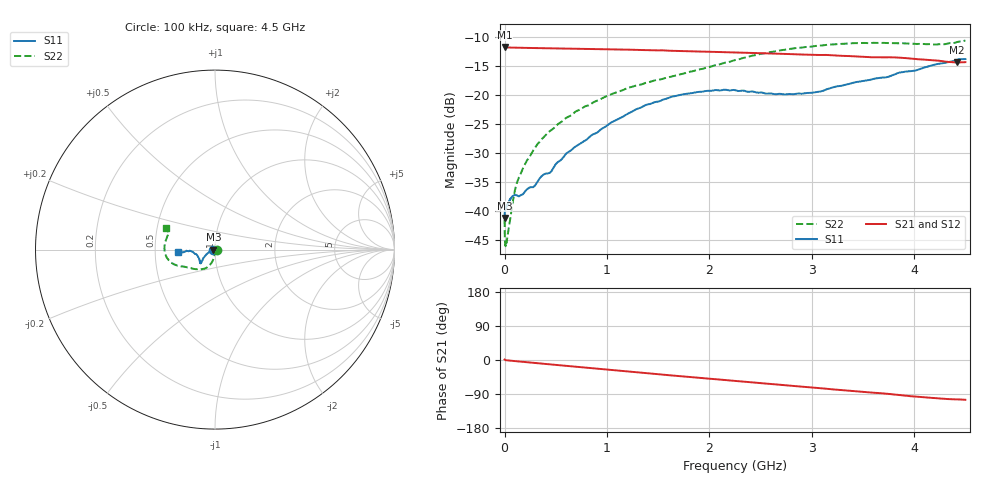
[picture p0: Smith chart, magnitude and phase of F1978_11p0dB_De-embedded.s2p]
! Integrated Device Technology
! Corporate Headquarters
! 6024 Silver Creek Valley Road
! San Jose, CA 95138  USA
! Phone:  1-408-284-8200
! Toll Free:  1-800-223-1366
! Webpage:  http://www.idt.com/
! Timing and RF Division
! 515 Groton Road, Suite 102
! Westford, MA 01886-6024
! Device:  F1978
! Description: 6-bit, 75 ohm, 0.5 dB Digital Step Attenuator
! Frequency:  5.0 MHz -  3.00 GHz
! Package:  4x4 mm QFN Plastic Package: 20 pin
! Ports:  2 RF, 11 DC
!  Pin  1  = D5 (16 dB)
!  Pin  2  = RF1  =  Port 1
!  Pin  3  = Serial Data In (DATA)
!  Pin  4  = Serial Clock (CLK)
!  Pin  5  = Serial Latch Enable (LE)
!  Pin  6  = VDD
!  Pin  7  = NC
!  Pin  8  = NC
!  Pin  9  = NC
!  Pin 10  = GND
!  Pin 11  = GND
!  Pin 12  = NC
!  Pin 13  = VMODE
!  Pin 14  = RF2  =  Port 2
!  Pin 15  = D4 (8 dB)
!  Pin 16  = D3 (4 dB)
!  Pin 17  = D2 (2 dB)
!  Pin 18  = NC
!  Pin 19  = D1 (1 dB)
!  Pin 20  = D0 (0.5 dB)
! State:  22
! Atten State:  11.0 dB
! Voltage:  +3.30 Volts
! Current:  0.592 mA
! Data:  The device was measured on a F1975 evaluation board which has
!  individual transmission lines to the RF pins.  Data was collected
!  using a calibrated network analyzer.  The evaluation board was
!  de-embedded using Automatic Fixture Removal (AFR).
!  The reference plane is the edge of the package pin.
! Misc:
!  Action Tracker AT0416
! Date Measured:  2018-02-08
! Date:  2018-03-26  MJV
! Note:
!  Integrated Device Technology supplies this data as a sample of measured
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# GHz S dB R 75
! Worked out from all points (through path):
!   291 points, 100 kHz to 4.5 GHz, reference 75 ohm
!   highest |S21| = -11.69 dB at 100 kHz (marker M1); lowest = -14.4 dB at 4.42 GHz (marker M2)
!   group delay of S21, straight-line fit = 66.3 ps
!   lowest |S11| = -41.1 dB at 100 kHz (marker M3), VSWR 1.02, Z = 73.7 - j0.00548 ohm
!   |S11| at or under -10 dB: start of sweep to end of sweep
!   |S22| runs from -46.0 to -10.6 dB; largest |S21 - S12| = 0.00015
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0.0001  -41.14 -179.8  -11.69 1.2  -11.69 1.2  -41.44 -2.6
0.0009  -40.29 -175.7  -11.72 1.0  -11.72 1.0  -43.85 -11.3
0.002  -39.96 -177.2  -11.73 0.8  -11.73 0.8  -44.74 -14.3
0.01  -39.47 -175.1  -11.76 -0.5  -11.76 -0.5  -45.98 -39.2
0.06  -37.73 -172.0  -11.80 -1.8  -11.80 -1.8  -40.71 -88.2
0.1  -37.15 -166.8  -11.82 -2.9  -11.82 -2.9  -36.44 -95.5
0.12  -37.25 -164.8  -11.83 -3.4  -11.83 -3.4  -35.08 -94.1
0.22  -36.17 -167.4  -11.86 -6.0  -11.86 -5.9  -31.18 -94.0
0.32  -34.94 -168.4  -11.89 -8.4  -11.89 -8.4  -28.44 -97.2
0.38  -33.66 -164.1  -11.91 -10.0  -11.91 -10.0  -27.26 -97.0
0.44  -33.39 -163.4  -11.92 -11.4  -11.92 -11.4  -26.20 -97.3
0.52  -31.50 -163.4  -11.95 -13.4  -11.94 -13.4  -25.00 -100.1
0.76  -28.09 -155.7  -12.01 -19.3  -12.01 -19.3  -22.21 -105.2
1.04  -24.70 -149.8  -12.10 -26.3  -12.09 -26.3  -19.85 -111.8
1.52  -20.99 -140.5  -12.28 -37.9  -12.27 -37.9  -17.29 -126.4
1.88  -19.46 -136.6  -12.47 -46.5  -12.47 -46.5  -15.65 -140.1
2.26  -19.18 -138.1  -12.65 -55.4  -12.64 -55.4  -13.93 -151.8
2.64  -19.83 -149.1  -12.84 -64.2  -12.84 -64.2  -12.46 -159.4
3.02  -19.53 -164.3  -13.05 -72.9  -13.05 -72.9  -11.57 -167.0
3.76  -16.76 -176.6  -13.48 -89.7  -13.47 -89.7  -11.03 174.0
4.42  -13.90 -174.7  -14.37 -104.0  -14.36 -104.0  -10.84 157.5
4.5  -13.78 -176.5  -14.31 -105.1  -14.31 -105.1  -10.58 156.2
